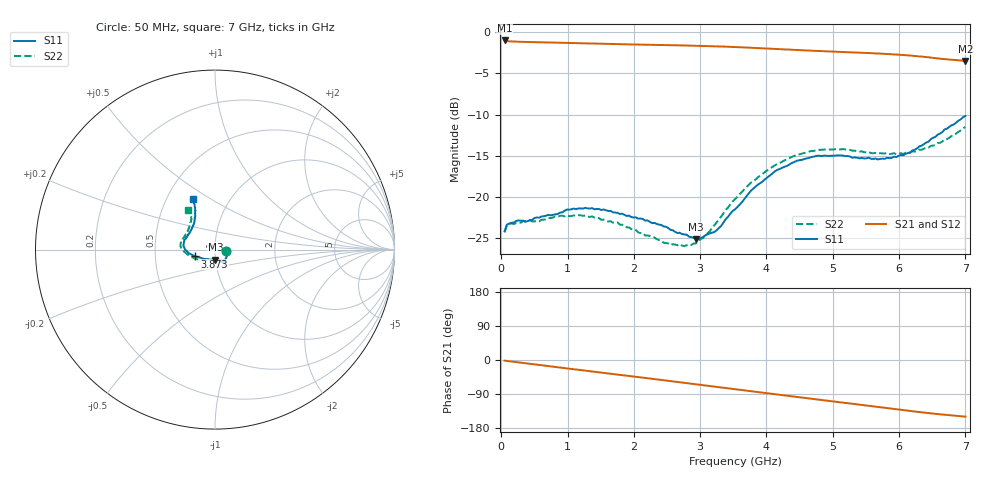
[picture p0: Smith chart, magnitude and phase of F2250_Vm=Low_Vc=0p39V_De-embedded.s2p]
! Integrated Device Technology
! Corporate Headquarters
! 6024 Silver Creek Valley Road
! San Jose, CA 95138  USA
! Phone:  1-408-284-8200
! Toll Free:  1-800-223-1366
! Webpage:  http://www.idt.com/
! Timing and RF Division
! 515 Groton Road, Suite 102
! Westford, MA 01886-6024
! Device:  F2250
! Description: Voltage Variable RF Attenuator
! Frequency:  50.0 -  6000.00 MHz
! Package:  3x3 mm Thin QFN Plastic Package: 16 pin
! Ports:  2 RF, 3 DC
!  Pin  1  = GND
!  Pin  2  = NC
!  Pin  3  = RF1  = Port 1
!  Pin  4  = NC
!  Pin  5  = GND
!  Pin  6  = GND
!  Pin  7  = GND
!  Pin  8  = GND
!  Pin  9  = NC
!  Pin 10  = RF2  = Port 2
!  Pin 11  = NC
!  Pin 12  = GND
!  Pin 13  = GND
!  Pin 14  = VCNTRL
!  Pin 15  = VDD
!  Pin 16  = VMODE
! Vcntrl:  0.390 Volts
! Vmode:  +0.000 Volts
! Vdd:  +3.30  Volts
! Current:  1.122 mA
! Data:  The device was measured on a the F2250 evaluation board which has
!  individual transmission lines to the RF pins.  Data was collected
!  using a calibrated network analyzer.  The evaluation board was
!  de-embedded using a TRL calibration technique.
!  The reference plane is the edge of the package pin.
! Misc:  SN 10
!  Action Tracker AT0258
! Date Measured:  2014-11-26
! Date:  2015-10-15  MJV
! Note:
!  Integrated Device Technology supplies this data as a sample of measured
!  data at the package pin for this product.  Your particular data for this
!  product may vary.
!  Data was taken at 25 degrees C.
!  Integrated Device Technology reserves the right to change this data at anytime.
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# GHz S dB R 50
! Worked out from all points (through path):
!   201 points, 50 MHz to 7 GHz, reference 50 ohm
!   highest |S21| = -0.99 dB at 50 MHz (marker M1); lowest = -3.5 dB at 7 GHz (marker M2)
!   group delay of S21, straight-line fit = 60 ps
!   lowest |S11| = -25.1 dB at 2.934 GHz (marker M3), VSWR 1.12, Z = 50 - j5.54 ohm
!   |S11| at or under -10 dB: start of sweep to end of sweep
!   |S22| runs from -26.0 to -11.5 dB; largest |S21 - S12| = 0.00034
!   S11 on the Smith chart (normalised r, x): 50 MHz: 1.13, -0.02; 3.873 GHz: 0.80, -0.06; 7 GHz: 0.67, +0.42
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0.05  -24.18 -8.8  -0.99 -1.8  -0.99 -1.8  -24.32 -9.5
0.08475  -23.37 -8.8  -1.06 -2.5  -1.06 -2.5  -23.47 -8.7
0.15425  -23.15 -10.9  -1.11 -4.0  -1.11 -4.0  -23.22 -10.5
0.57125  -22.53 -28.1  -1.21 -13.1  -1.21 -13.1  -22.97 -29.3
0.71025  -22.19 -35.9  -1.24 -16.2  -1.24 -16.2  -22.55 -37.2
1.2315  -21.43 -53.1  -1.35 -27.4  -1.35 -27.4  -22.31 -58.0
1.75275  -21.94 -59.8  -1.44 -38.4  -1.44 -38.4  -23.11 -65.8
2.37825  -23.37 -61.0  -1.53 -51.8  -1.53 -51.8  -25.25 -69.1
2.552  -24.01 -64.9  -1.56 -55.6  -1.56 -55.6  -25.86 -74.8
2.83  -24.83 -78.9  -1.61 -61.7  -1.61 -61.7  -25.99 -93.0
2.93425  -25.15 -87.2  -1.63 -64.0  -1.63 -64.0  -25.67 -101.3
3.21225  -24.28 -116.0  -1.69 -70.2  -1.69 -70.2  -23.46 -126.1
3.525  -21.52 -143.8  -1.79 -77.1  -1.79 -77.1  -20.29 -145.1
3.8725  -18.49 -161.2  -1.92 -84.8  -1.92 -84.8  -17.61 -160.6
4.1505  -16.77 -171.3  -2.03 -90.9  -2.03 -90.9  -16.06 -170.6
4.4285  -15.73 -179.1  -2.14 -96.9  -2.14 -96.9  -14.99 -177.8
4.7065  -15.12 174.1  -2.24 -102.9  -2.24 -102.9  -14.43 176.1
5.15825  -14.99 163.3  -2.40 -112.6  -2.40 -112.6  -14.19 166.9
5.85325  -15.30 140.0  -2.65 -127.6  -2.65 -127.6  -14.79 151.6
6.166  -14.61 128.8  -2.82 -134.4  -2.82 -134.4  -14.62 142.7
6.444  -13.30 120.3  -3.03 -140.2  -3.03 -140.2  -14.02 133.3
7  -10.16 113.7  -3.47 -149.5  -3.47 -149.5  -11.51 123.9
